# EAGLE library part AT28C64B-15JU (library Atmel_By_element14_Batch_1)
64K Parallel EEPROM
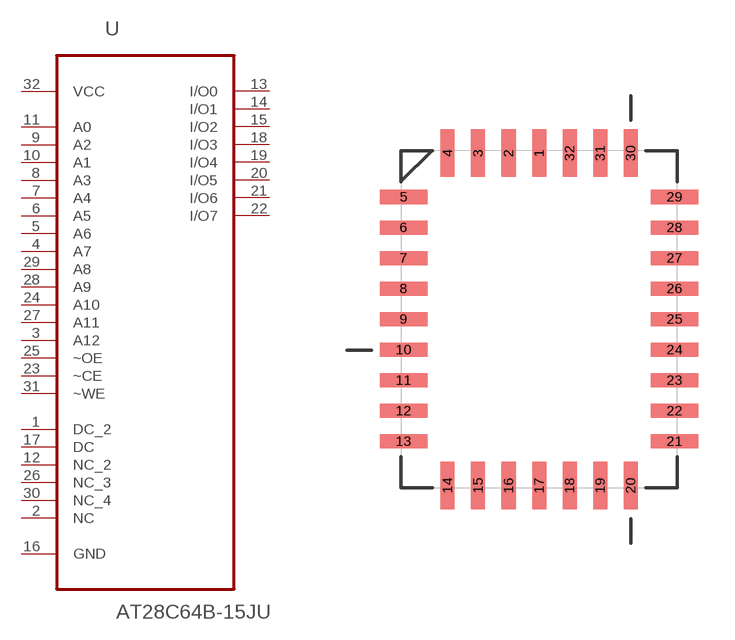
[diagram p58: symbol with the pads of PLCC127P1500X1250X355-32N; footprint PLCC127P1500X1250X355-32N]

Designator prefix U

## AT28C64B-15JU (DESCRIPTION: 64K Parallel EEPROM; MPN: AT28C64B-15JU; OC_FARNELL: 1095783; OC_NEWARK: 96K6556; PACKAGE: PLCC-32; SUPPLIER: Atmel)  [PLCC127P1500X1250X355-32N]
1  DC_2  nc
2  NC  nc
3  A12  in
4  A7  in
5  A6  in
6  A5  in
7  A4  in
8  A3  in
9  A2  in
10  A1  in
11  A0  in
12  NC_2  nc
13  I/O0  out
14  I/O1  out
15  I/O2  out
16  GND  pas
17  DC  nc
18  I/O3  out
19  I/O4  out
20  I/O5  out
21  I/O6  out
22  I/O7  out
23  ~CE  in
24  A10  in
25  ~OE  in
26  NC_3  nc
27  A11  in
28  A9  in
29  A8  in
30  NC_4  nc
31  ~WE  in
32  VCC  pwr

## Footprint PLCC127P1500X1250X355-32N (pad centres in mm)
smd 0.584 x 1.981: 1 0,6.909; 2 -1.27,6.909; 3 -2.54,6.909; 4 -3.81,6.909; 14 -3.81,-6.909; 15 -2.54,-6.909; 16 -1.27,-6.909; 17 0,-6.909; 18 1.27,-6.909; 19 2.54,-6.909; 20 3.81,-6.909; 30 3.81,6.909; 31 2.54,6.909; 32 1.27,6.909
smd 1.981 x 0.584: 5 -5.639,5.08; 6 -5.639,3.81; 7 -5.639,2.54; 8 -5.639,1.27; 9 -5.639,0; 10 -5.639,-1.27; 11 -5.639,-2.54; 12 -5.639,-3.81; 13 -5.639,-5.08; 21 5.639,-5.08; 22 5.639,-3.81; 23 5.639,-2.54; 24 5.639,-1.27; 25 5.639,0; 26 5.639,1.27; 27 5.639,2.54; 28 5.639,3.81; 29 5.639,5.08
